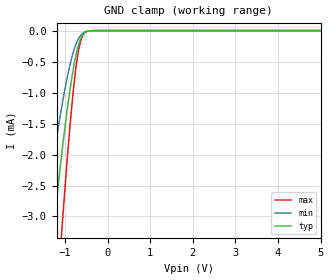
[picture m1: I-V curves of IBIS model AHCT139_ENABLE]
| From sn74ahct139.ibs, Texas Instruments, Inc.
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[Model]   AHCT139_ENABLE
Model_type  Input
Vinl = 0.8
Vinh = 2.0
| variable   typ   min   max
C_comp   0.76pF   0.58pF   0.87pF
[Temperature Range]   40   100   -40
| Ambient temperature   25   85   -40
[Voltage range]   5   4.5   5.5
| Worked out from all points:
|   GND clamp passes 1 mA (typ) near -0.89 V on its own axis
[GND Clamp]
| AHCT139_ENABLE
|   Voltage   I(typ)   I(min)   I(max)
-5V       -39.32mA   -26.22mA   -50.69mA
-1.54V    -5.159mA   -3.345mA   -8.051mA
-1.49V    -4.782mA   -3.093mA   -7.502mA
-1.28V    -3.281mA   -2.092mA   -5.261mA
-1.25V    -3.08mA    -1.957mA   -4.951mA
-1.08V    -2.006mA   -1.239mA   -3.266mA
-900mV    -1.033mA   -600.8uA   -1.67mA
-775mV    -505.6uA   -279.7uA   -774.7uA
-720mV    -329uA     -181uA     -476.3uA
-660mV    -182.6uA   -103.6uA   -241uA
-540mV    -34.72uA   -24.11uA   -34.5uA
5V        17.64nA    1.142nA    163.4nA
